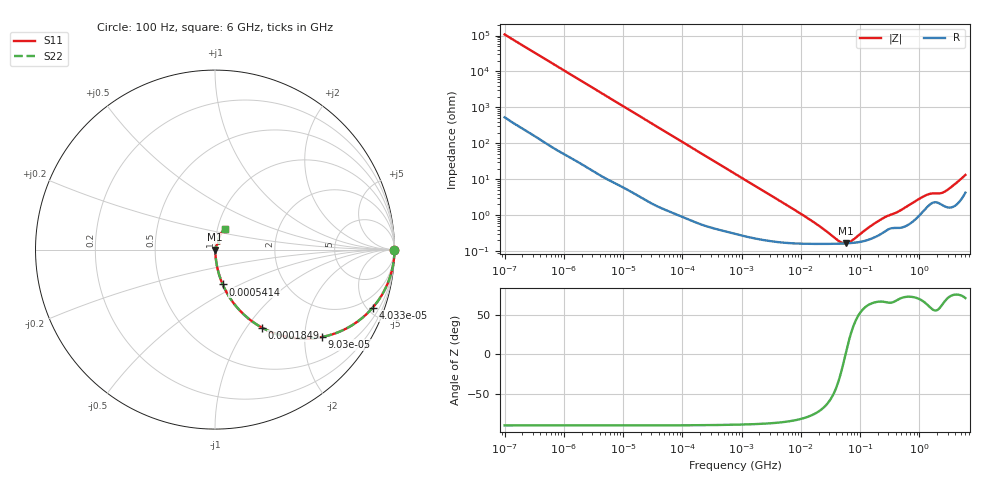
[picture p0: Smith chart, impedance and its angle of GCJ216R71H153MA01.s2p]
!Murata Part Number: GCJ216R71H153MA01
!These Parameters are Measured in Series Mode Connection
!Data Generated on Mar 13, 2026
!  o--ll--o
!Port1  Port2
!  o------o
!Operation Temp=25[degC], DC Bias Voltage=0[V]
!Freq. Start=100[Hz] Stop=6[GHz] 401[Steps]
# Hz S RI R 50
!Freq.(Hz) S11(Real) S11(Imag) S21(Real) S21(Imag) S12(Real) S12(Imag) S22(Real) S22(Imag)
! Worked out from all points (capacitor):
!   401 points, 100 Hz to 6 GHz, reference 50 ohm
!   read as one part in series: C = 14.8 nF near 109 Hz
!   lowest |Z| = 165 mohm at 56.99 MHz (marker M1)
!   series resonance near 56.77 MHz, so ESL is about 530 pH
!   S11 on the Smith chart (normalised r, x): 100 Hz: open; 40.34 kHz: 1.03, -5.41; 90.3 kHz: 1.02, -2.42; 184.9 kHz: 1.01, -1.19; 541.4 kHz: 1.01, -0.41; 6 GHz: 1.09, +0.25
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100  1 -0.000933  5.5e-06 0.000933  5.5e-06 0.000933  1 -0.000933
2008  0.9996 -0.0186  0.000436 0.0186  0.000436 0.0186  0.9996 -0.0186
11514  0.9883 -0.1047  0.0117 0.1047  0.0117 0.1047  0.9883 -0.1047
23569  0.9542 -0.2062  0.0458 0.2062  0.0458 0.2062  0.9542 -0.2062
40335  0.8782 -0.3239  0.1218 0.3239  0.1218 0.3239  0.8782 -0.3239
60352  0.7646 -0.4207  0.2354 0.4207  0.2354 0.4207  0.7646 -0.4207
90302  0.5942 -0.4871  0.4058 0.4871  0.4058 0.4871  0.5942 -0.4871
184852  0.2628 -0.4352  0.7372 0.4352  0.7372 0.4352  0.2628 -0.4352
302498  0.1199 -0.3186  0.8801 0.3186  0.8801 0.3186  0.1199 -0.3186
541393  0.043 -0.1944  0.957 0.1944  0.957 0.1944  0.043 -0.1944
774597  0.0229 -0.1392  0.9771 0.1392  0.9771 0.1392  0.0229 -0.1392
2481164  0.00401 -0.0447  0.996 0.0447  0.996 0.0447  0.00401 -0.0447
1.555665e7  0.00164 -0.00667  0.9984 0.00667  0.9984 0.00667  0.00164 -0.00667
4.35672e7  0.00162 -0.00106  0.9984 0.00106  0.9984 0.00106  0.00162 -0.00106
5.699437e7  0.00165 1.59e-05  0.9984 -1.59e-05  0.9984 -1.59e-05  0.00165 1.59e-05
7.129496e7  0.00169 0.00091  0.9983 -0.00091  0.9983 -0.00091  0.00169 0.00091
1.596157e8  0.00229 0.00481  0.9977 -0.00481  0.9977 -0.00481  0.00229 0.00481
3.124326e8  0.00425 0.00905  0.9957 -0.00905  0.9957 -0.00905  0.00425 0.00905
4.470121e8  0.00455 0.0119  0.9954 -0.0119  0.9954 -0.0119  0.00455 0.0119
1.309207e9  0.0167 0.0317  0.9833 -0.0317  0.9833 -0.0317  0.0167 0.0317
2.679998e9  0.019 0.0403  0.981 -0.0403  0.981 -0.0403  0.019 0.0403
6e9  0.0546 0.114  0.9454 -0.114  0.9454 -0.114  0.0546 0.114
